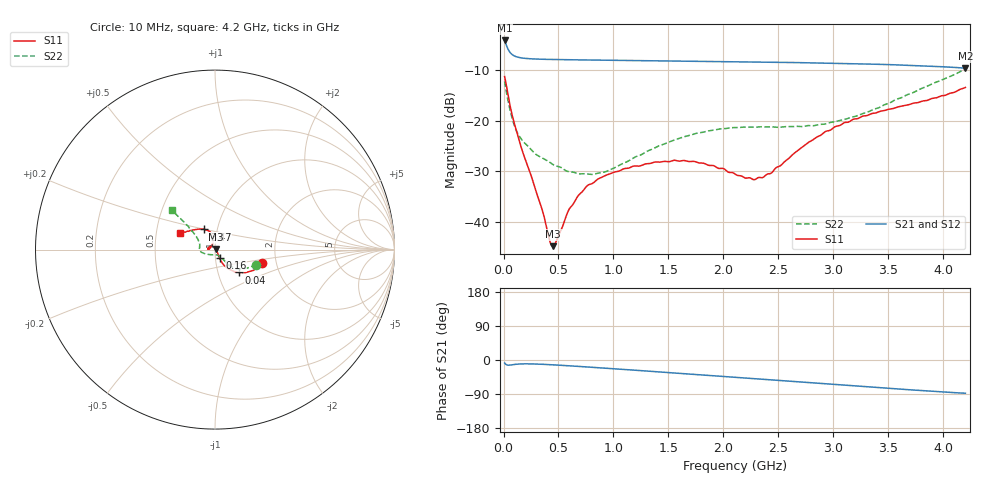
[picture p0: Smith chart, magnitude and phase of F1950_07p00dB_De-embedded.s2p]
! Integrated Device Technology
! Corporate Headquarters
! 6024 Silver Creek Valley Road
! San Jose, CA 95138  USA
! Phone:  1-408-284-8200
! Toll Free:  1-800-223-1366
! Webpage:  http://www.idt.com/
! Timing and RF Division
! 515 Groton Road, Suite 102
! Westford, MA 01886-6024
! Device:  F1950
! Description: 7-bit 0.25 dB Digital Step Attenuator
! Frequency:  150.0 -  4000.00 MHz
! Package:  4x4 mm Thin QFN Plastic Package: 24 pin
! Ports:  2 RF, 12 DC
!  Pin  1  = D0
!  Pin  2  = VDD
!  Pin  3  = Vmode
!  Pin  4  = GND
!  Pin  5  = RF1  =  Port 1
!  Pin  6  = GND
!  Pin  7  = GND
!  Pin  8  = GND
!  Pin  9  = GND
!  Pin 10  = GND
!  Pin 11  = GND
!  Pin 12  = GND
!  Pin 13  = GND
!  Pin 14  = RF2  =  Port 2
!  Pin 15  = GND
!  Pin 16  = LE
!  Pin 17  = CLK
!  Pin 18  = DATE
!  Pin 19  = D6
!  Pin 20  = D5
!  Pin 21  = D4
!  Pin 22  = D3
!  Pin 23  = D2
!  Pin 24  = D1
! State:  28
! Atten State:  7.00 dB
! Voltage:  +5.00 Volts
! Current:  Not Measured mA
! Data:  The device was measured on a the F195X evaluation board which has
!  individual transmission lines to the RF pins.  Data was collected
!  using a calibrated network analyzer.  The evaluation board was
!  de-embedded using a TRL calibration technique.
!  The reference plane is the edge of the package pin.
! Misc:  Board 2019
!  Action Tracker AT0250
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# GHz S dB R 50
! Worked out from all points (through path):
!   420 points, 10 MHz to 4.2 GHz, reference 50 ohm
!   highest |S21| = -4.07 dB at 10 MHz (marker M1); lowest = -9.6 dB at 4.2 GHz (marker M2)
!   group delay of S21, straight-line fit = 55.4 ps
!   lowest |S11| = -44.9 dB at 450 MHz (marker M3), VSWR 1.01, Z = 50.5 + j0.262 ohm
!   |S11| at or under -10 dB: start of sweep to end of sweep
!   |S22| runs from -30.6 to -9.8 dB; largest |S21 - S12| = 0.00053
!   S11 on the Smith chart (normalised r, x): 10 MHz: 1.69, -0.28; 40 MHz: 1.26, -0.33; 160 MHz: 1.05, -0.10; 3.47 GHz: 0.87, +0.20; 4.2 GHz: 0.67, +0.13
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0.01  -11.22 -16.2  -4.07 -8.0  -4.07 -8.0  -12.20 -20.1
0.04  -14.73 -44.0  -5.74 -13.6  -5.74 -13.7  -15.92 -41.6
0.1  -20.64 -60.9  -7.16 -11.7  -7.15 -11.7  -21.01 -49.3
0.16  -25.20 -61.8  -7.52 -10.4  -7.52 -10.4  -23.57 -51.5
0.35  -37.50 -38.0  -7.80 -11.3  -7.80 -11.3  -27.32 -57.1
0.42  -43.76 -3.4  -7.83 -12.3  -7.83 -12.3  -28.22 -58.8
0.45  -44.85 26.9  -7.85 -12.7  -7.85 -12.7  -28.67 -61.3
0.48  -43.86 56.9  -7.86 -13.2  -7.86 -13.2  -28.95 -64.2
0.59  -37.82 102.4  -7.89 -15.2  -7.89 -15.2  -30.06 -72.6
0.71  -34.19 117.9  -7.93 -17.4  -7.93 -17.4  -30.51 -85.5
0.77  -32.72 122.3  -7.94 -18.6  -7.94 -18.6  -30.57 -92.4
0.94  -30.72 135.4  -7.99 -21.9  -7.99 -21.9  -29.98 -114.8
1.41  -28.19 164.5  -8.11 -31.3  -8.11 -31.3  -24.99 -154.1
1.74  -28.08 176.5  -8.19 -38.0  -8.19 -38.1  -22.56 -167.1
2.11  -30.61 167.8  -8.29 -45.7  -8.29 -45.8  -21.36 -177.6
2.27  -31.65 146.8  -8.34 -49.0  -8.34 -49.0  -21.26 178.4
2.36  -31.22 132.2  -8.37 -50.9  -8.37 -50.9  -21.17 176.1
2.81  -23.82 99.0  -8.51 -60.3  -8.51 -60.3  -20.98 161.3
3.1  -20.35 104.2  -8.63 -66.4  -8.63 -66.4  -19.73 152.4
3.47  -17.93 117.8  -8.84 -74.1  -8.84 -74.1  -16.76 142.9
3.51  -17.67 119.6  -8.86 -74.9  -8.86 -74.9  -16.48 142.2
4.2  -13.38 154.2  -9.57 -87.7  -9.56 -87.8  -9.79 137.7
